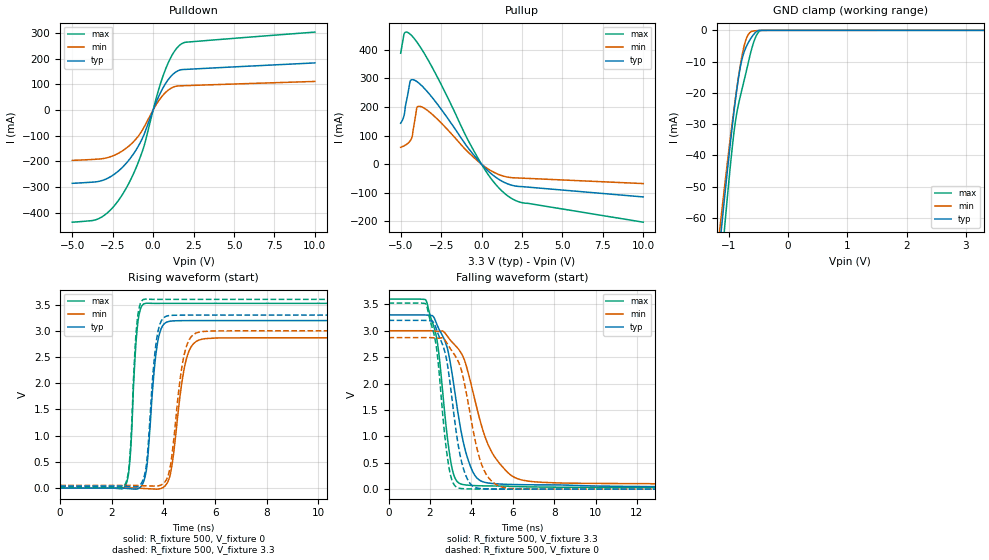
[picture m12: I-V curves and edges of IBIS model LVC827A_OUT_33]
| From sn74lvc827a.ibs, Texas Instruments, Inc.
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[Model]   LVC827A_OUT_33
Model_type  3-state
Enable   Active-Low
Vref =   0
Rref =   500
Cref =   50p
Vmeas =   1.5
| variable   typ   min   max
C_comp   5.75pF   5.10pF   6.89pF
| C_pullup   7.52pF   6.21pF   8.53pF
| C_pulldown   10.56pF   6.95pF   16.57pF
| C_tri-state   5.75pF   5.10pF   6.89pF
[Temperature Range]   40   100   -40
| Ambient temperature   25   85   -40
[Voltage range]   3.3   3   3.6
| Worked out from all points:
|   slope of the pulldown table from 0 to 0.495 V, typ, clamps not added: 6.81 ohm
|   slope of the pullup table from 0 to 0.495 V, typ, clamps not added: 17.6 ohm
|   GND clamp passes 1 mA (typ) near -0.57 V on its own axis
|   rising waveform, R_fixture 500, V_fixture 0: 20-80 % time 307ps typ, 440ps min, 217ps max; typ from 0 V to 3.19 V
|   falling waveform, R_fixture 500, V_fixture 3.3: 20-80 % time 885ps typ, 1.38ns min, 609ps max; typ from 3.3 V to 0.039 V
|   rising waveform, R_fixture 500, V_fixture 3.3: 20-80 % time 296ps typ, 418ps min, 210ps max; typ from 0.039 V to 3.3 V
|   falling waveform, R_fixture 500, V_fixture 0: 20-80 % time 711ps typ, 920ps min, 552ps max; typ from 3.2 V to 0 V
[GND Clamp]
| LVC827A_OUT_33
|   Voltage   I(typ)   I(min)   I(max)
-5V       -931.5mA   -844.2mA   -1.078A
-1.145V   -67.43mA   -62.49mA   -79.41mA
-1.11V    -60.81mA   -56.56mA   -71.73mA
-1.075V   -54.3mA    -50.72mA   -64.17mA
-1.045V   -48.81mA   -45.79mA   -57.83mA
-905mV    -24.96mA   -24.22mA   -31.61mA
-795mV    -10.82mA   -10.09mA   -20.28mA
-735mV    -6.635mA   -4.578mA   -15.56mA
-680mV    -4.289mA   -1.644mA   -11.12mA
-575mV    -1.197mA   -182.8uA   -3.545mA
-475mV    -13.49uA   -55.9uA    -163uA
3.3V      82.23pA    54.45nA    -1.069nA
[Pulldown]
| LVC827A_OUT_33
|   Voltage   I(typ)   I(min)   I(max)
-5V       -286mA     -196.5mA   -437.6mA
-3.21V    -276.2mA   -190.6mA   -418.6mA
-2.515V   -255.5mA   -179.5mA   -381.7mA
-1.825V   -218.9mA   -156.4mA   -322.2mA
-1.205V   -170.3mA   -123.2mA   -247.1mA
-640mV    -106.8mA   -75.79mA   -156.2mA
235mV     37.25mA    25.43mA    56.34mA
730mV     99.32mA    65.88mA    153mA
1.205V    138mA      88mA       217.5mA
1.675V    156.1mA    94.11mA    254.3mA
2.035V    158.3mA    94.92mA    264.3mA
10V       183.5mA    111.3mA    303.7mA
[Pullup]
| LVC827A_OUT_33
|   Voltage   I(typ)   I(min)   I(max)
-5V       143.4mA    58.9mA     387.9mA
-4.735V   189.8mA    65.84mA    460mA
-4.415V   289.4mA    81.4mA     454.6mA
-4.28V    295.5mA    98.7mA     447mA
-4.085V   291.9mA    167.2mA    433.6mA
-3.955V   287mA      200.9mA    423.6mA
-3.49V    262.2mA    193.8mA    382.4mA
-35mV     2.231mA    1.61mA     3.344mA
825mV     -43.35mA   -30.08mA   -67.18mA
1.685V    -70.13mA   -45.81mA   -113.3mA
2.55V     -78.57mA   -48.86mA   -135mA
10V       -114.4mA   -67.74mA   -202.7mA
[Ramp]
| LVC827A_OUT_33
| variable   typ   min   max
dV/dt_r   1.93/3.20E-10   1.73/4.49E-10   2.12/2.24E-10
dV/dt_f   1.96/8.86E-10   1.77/1.39E-09   2.14/6.11E-10
R_load = 500
[Rising Waveform]
| LVC827A_OUT_33
R_fixture =   500
C_fixture =   0
L_fixture =   0
V_fixture =   0
V_fixture_min = 0
V_fixture_max = 0
|   Time   V(typ)   V(min)   V(max)
0s        540.1pV    2.024nV    13.49nV
2.535ns   -5.245mV   1.205mV    53.44mV
2.715ns   -13.05mV   1.279mV    626.9mV
3ns       -13.82mV   -1.793mV   3.122V
3.325ns   305.6mV    -10.16mV   3.526V
3.765ns   2.756V     -20.54mV   3.523V
4.29ns    3.185V     325.7mV    3.524V
4.88ns    3.194V     2.45V      3.524V
5.625ns   3.195V     2.851V     3.524V
50ns      3.195V     2.866V     3.524V
[Falling Waveform]
| LVC827A_OUT_33
R_fixture =   500
C_fixture =   0
L_fixture =   0
V_fixture =   3.3
V_fixture_min = 3
V_fixture_max = 3.6
|   Time   V(typ)   V(min)   V(max)
0s        3.3V       3V         3.6V
1.83ns    3.298V     3V         3.561V
2.36ns    3.098V     2.99V      2.775V
2.805ns   2.716V     2.917V     1.104V
3.05ns    2.236V     2.793V     429.8mV
3.615ns   886.4mV    2.496V     86.34mV
4.17ns    261.1mV    1.693V     67.39mV
4.935ns   110.7mV    739.4mV    60.66mV
6.735ns   83.46mV    152.6mV    43.54mV
50ns      38.94mV    51.44mV    28.29mV
[Rising Waveform]
| LVC827A_OUT_33
R_fixture =   500
C_fixture =   0
L_fixture =   0
V_fixture =   3.3
V_fixture_min = 3
V_fixture_max = 3.6
|   Time   V(typ)   V(min)   V(max)
0s        38.92mV    51.28mV    28.29mV
2.535ns   33.83mV    52.35mV    89.14mV
2.705ns   27.64mV    52.35mV    643mV
2.985ns   29.32mV    49.61mV    3.205V
3.295ns   315.1mV    43.12mV    3.605V
3.73ns    2.823V     38.68mV    3.599V
4.21ns    3.29V      291.1mV    3.6V
4.815ns   3.299V     2.572V     3.6V
5.505ns   3.3V       2.986V     3.6V
50ns      3.3V       3V         3.6V
[Falling Waveform]
| LVC827A_OUT_33
R_fixture =   500
C_fixture =   0
L_fixture =   0
V_fixture =   0
V_fixture_min = 0
V_fixture_max = 0
|   Time   V(typ)   V(min)   V(max)
0s        3.197V     2.87V      3.525V
1.83ns    3.194V     2.87V      3.486V
2.315ns   3.026V     2.863V     2.685V
2.745ns   2.564V     2.813V     911.6mV
3.035ns   1.81V      2.633V     207.1mV
3.425ns   707.8mV    2.365V     17.52mV
3.875ns   143.6mV    1.571V     5.037mV
4.52ns    9.21mV     444mV      2.034mV
5.745ns   2.017mV    18.72mV    1.35mV
50ns      15.19uV    62.67uV    4.599uV
